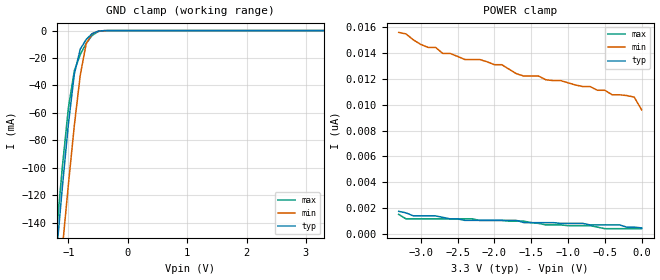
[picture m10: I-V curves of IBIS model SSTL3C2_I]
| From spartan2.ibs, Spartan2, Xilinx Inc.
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|   Model SSTL3C2_I
[Model]   SSTL3C2_I
Model_type   Input
Polarity   Non-Inverting
Vinl =   1.300V
Vinh =   1.700V
C_comp   6.5000pF   5.0000pF   8.0000pF
[Temperature Range]   27.0000   100.0000   0.000
[Voltage Range]   3.3000V   3.0000V   3.6000V
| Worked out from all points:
|   GND clamp passes 1 mA (typ) near -0.53 V on its own axis
[GND_clamp]
| voltage   I(typ)   I(min)   I(max)
-3.3V     -1.286A    -1.272A    -1.289A
-1.2V     -161.8mA   -205.3mA   -146.7mA
-1.1V     -113.2mA   -157.8mA   -98.56mA
-1V       -68.04mA   -112mA     -56.27mA
-900mV    -31.6mA    -69.09mA   -29.2mA
-800mV    -13.5mA    -32.34mA   -17.42mA
-700mV    -6.408mA   -9.455mA   -9.303mA
-600mV    -2.237mA   -2.349mA   -3.538mA
-500mV    -423.5uA   -545.3uA   -698.3uA
-400mV    -42.44uA   -91.26uA   -59.96uA
3.3V      465.7pA    10.83nA    27.36nA
[POWER_clamp]
| voltage   I(typ)   I(min)   I(max)
-3.3V     1.746nA    15.6nA     1.513nA
-3.2V     1.63nA     15.48nA    1.164nA
-3V       1.397nA    14.67nA    1.164nA
-2.8V     1.397nA    14.44nA    1.164nA
-2.7V     1.281nA    13.97nA    1.164nA
-1.9V     1.048nA    13.1nA     1.048nA
-1.6V     873.1pA    12.22nA    989.5pA
-1.4V     873.1pA    12.22nA    814.9pA
-700mV    698.5pA    11.41nA    640.3pA
-400mV    698.5pA    10.77nA    407.5pA
-100mV    523.9pA    10.59nA    407.5pA
0V        465.7pA    9.604nA    407.5pA
